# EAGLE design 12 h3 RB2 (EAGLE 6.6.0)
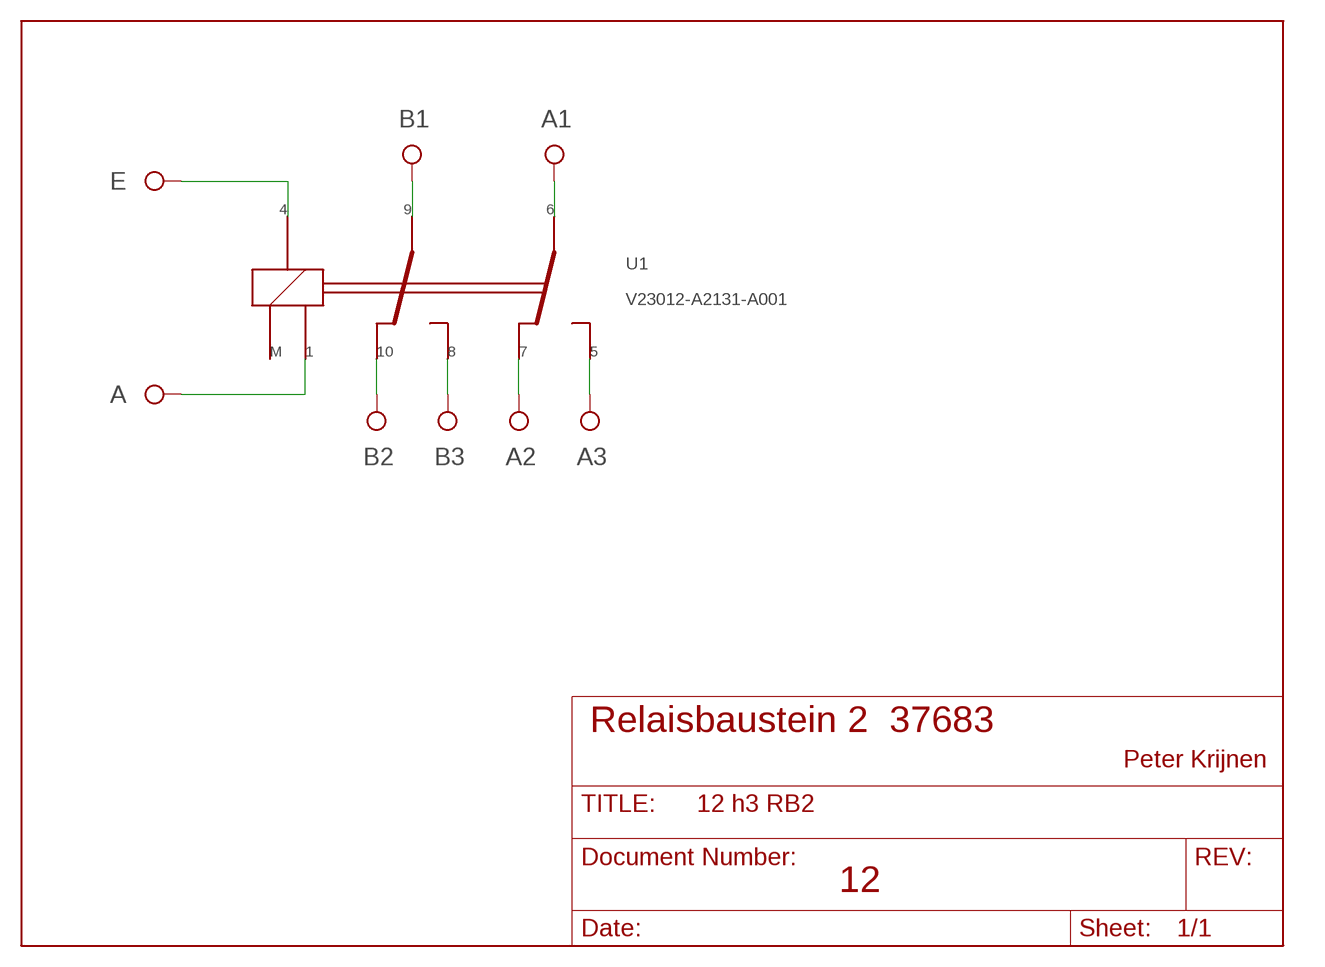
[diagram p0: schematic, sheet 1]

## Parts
A  PIN_2  [PIN_2]
A1  PIN_2  [PIN_2]
A2  PIN_2  [PIN_2]
A3  PIN_2  [PIN_2]
B1  PIN_2  [PIN_2]
B2  PIN_2  [PIN_2]
B3  PIN_2  [PIN_2]
E  PIN_2  [PIN_2]
U1  V23012-A2131-A001  V23012-A2131  [V23012]

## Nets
N$1: B2.P$1 U1.10
N$2: B3.P$1 U1.8
N$3: A2.P$1 U1.7
N$4: A3.P$1 U1.5
N$5: A1.P$1 U1.6
N$6: B1.P$1 U1.9
N$9: A.P$1 U1.1
N$12: E.P$1 U1.4
Unconnected: U1.M

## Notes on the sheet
- Relaisbaustein 2  37683
- Peter Krijnen
- 12

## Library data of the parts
A A1-A3 B1-B3 E = ft_spec:PIN_2
U1 = FT-SPEC:V23012

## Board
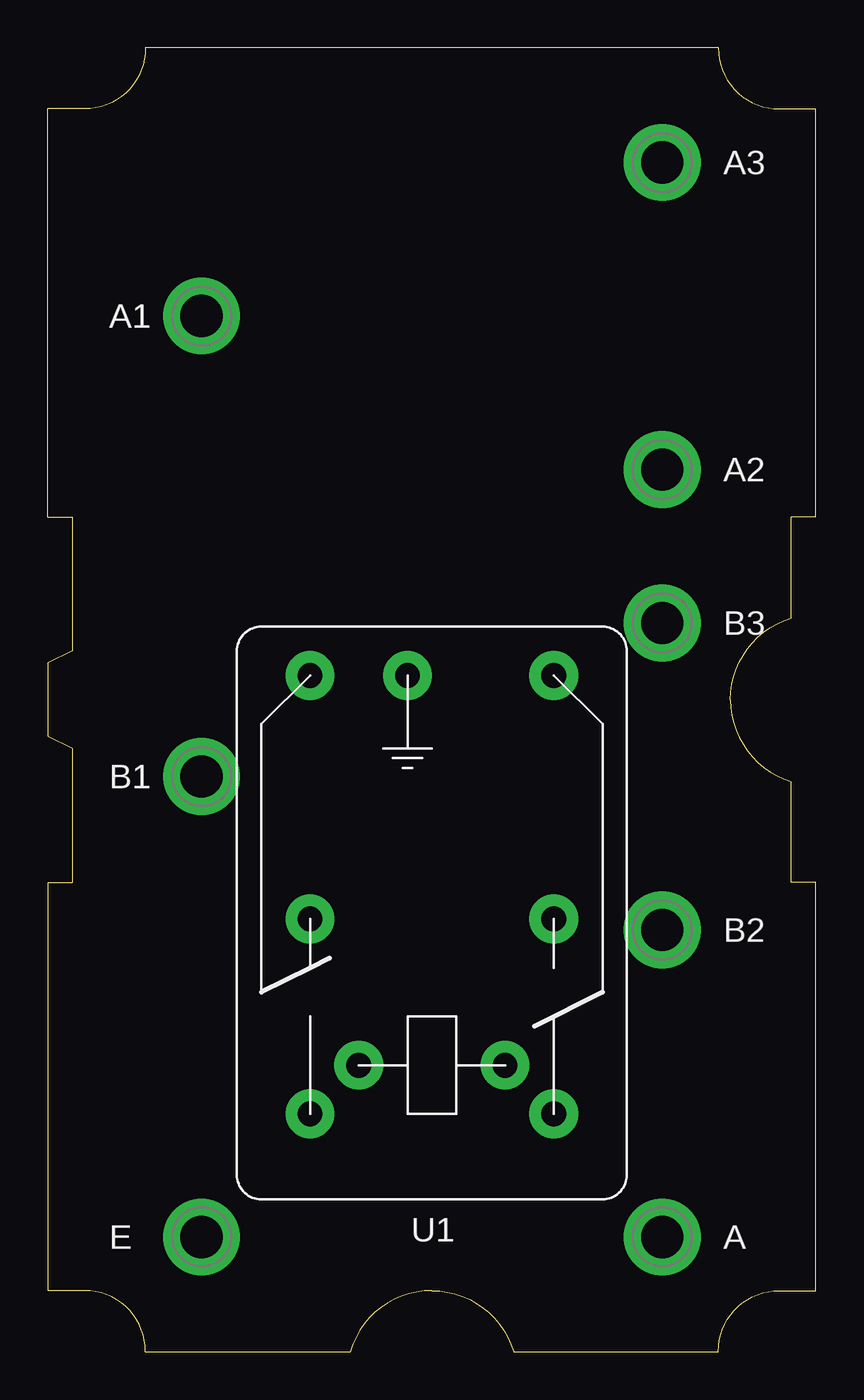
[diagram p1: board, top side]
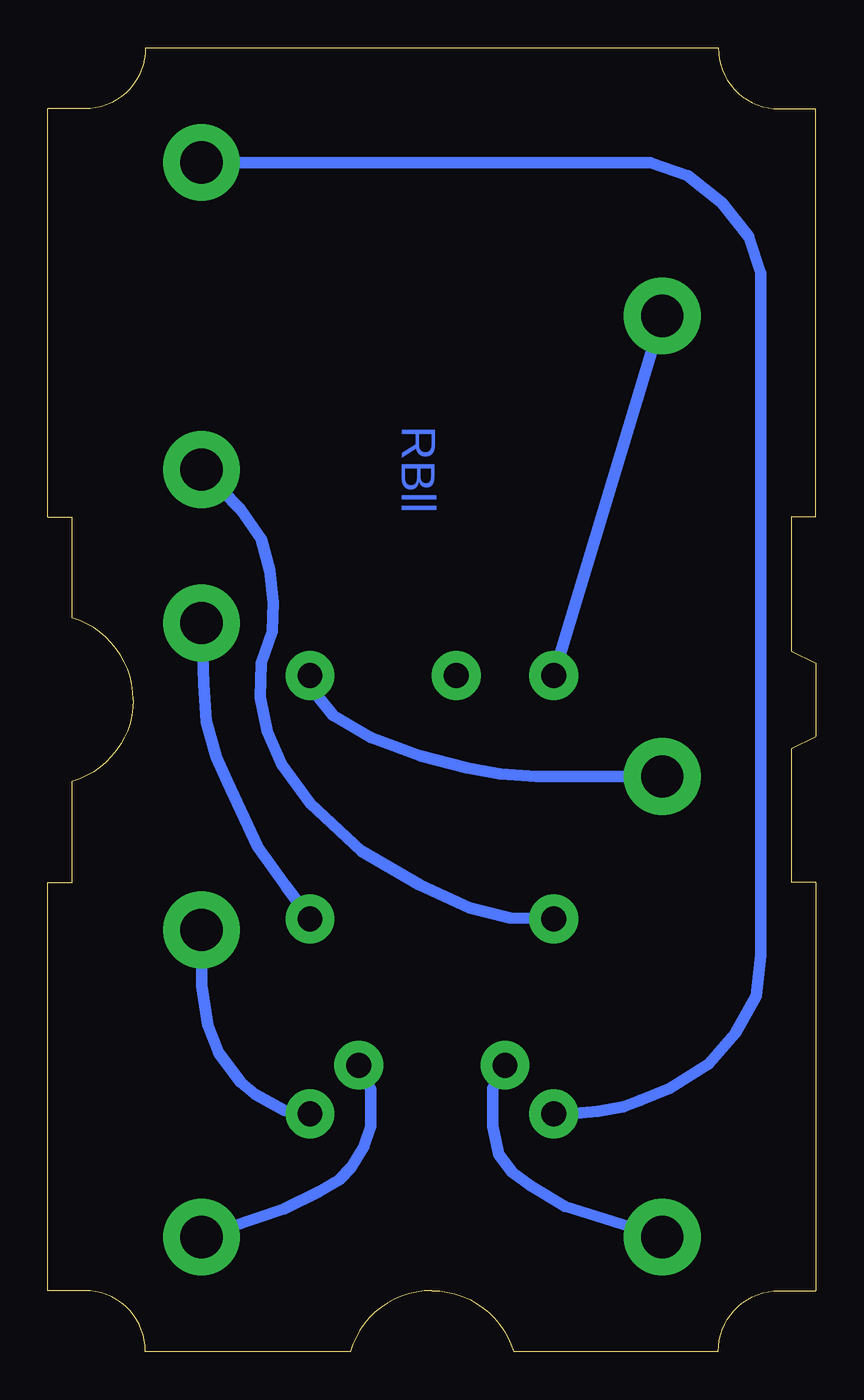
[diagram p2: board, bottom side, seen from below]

Size 40.01 x 67.94 mm. Coordinates in mm from the lower left corner, seen from the top.
Copper layers 16: Bottom 0.035mm
Design rules "default": minimum track width 10mil, minimum drill 24mil, track to track 8mil, track to pad 8mil, pad to pad 8mil, via to via 8mil, smd to smd 8mil, copper to edge 0.25mm, drill to drill 8mil, minimum pad ring 10mil, minimum via ring 8mil, stop-mask expansion 0mil, vias tented up to drill 0mil, thermal gap 10mil

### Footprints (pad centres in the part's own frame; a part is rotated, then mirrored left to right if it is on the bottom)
PIN_2 = drill 2.2 pad 4: P$1 0,0
V23012 = drill 1.3 pad 2.54: 1 -7.62,-3.81; 4 -7.62,3.81; 5 -10.16,6.35; 6 12.7,6.35; 7 0,6.35; 8 0,-6.35; 9 12.7,-6.35; 10 -10.16,-6.35; M 12.7,1.27

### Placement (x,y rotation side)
A  32,5.97 0 top
A1  8,53.98 0 top
A2  32,45.97 0 top
A3  32,61.98 0 top
B1  8,29.97 0 top
B2  32,21.97 0 top
B3  32,37.97 0 top
E  8,5.97 0 top
U1  20,22.54 90 top
U$1  [PRINTFORM_4575]  40.01,0 90 top
U$2  [DIM_4070]  40.01,0 90 top

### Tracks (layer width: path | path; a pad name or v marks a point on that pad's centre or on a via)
N$1
  Bottom 0.61: U1.10 27.69,12.57 29.21,13.4 29.97,14.03 31.11,15.56 31.69,17.02 32,19.05 B2.P$1
N$2
  Bottom 0.61: U1.8 27.62,24.26 29.08,26.29 30.67,29.72 31.24,30.99 31.75,32.83 31.88,34.8 B3.P$1
N$3
  Bottom 0.61: U1.7 15.94,22.61 18.03,23.11 20.64,24.32 23.69,26.1 26.35,28.57 27.81,30.61 28.57,32.32 28.96,34.1 28.89,35.88 28.32,37.53 28.26,39.05 28.45,40.7 28.89,42.35 29.97,43.88 A2.P$1
N$4
  Bottom 0.61: U1.5 12.26,12.45 11.37,12.51 10.03,12.76 9.14,13.08 7.62,13.72 5.59,14.99 4.19,16.57 3.11,18.54 2.86,20.64 2.86,56.2 3.49,58.1 4.89,59.88 6.67,61.28 8.64,61.98 A3.P$1
N$5
  Bottom 0.61: U1.6 A1.P$1
N$6
  Bottom 0.61: U1.9 25.91,34.1 25.15,33.15 23.18,32 20.57,31.05 18.16,30.42 16.45,30.1 14.54,29.97 B1.P$1
N$9
  Bottom 0.61: U1.1 23.18,13.65 23.18,11.75 23.56,10.67 24.19,9.59 24.83,8.95 25.91,8.32 27.69,7.43 A.P$1
N$12
  Bottom 0.61: U1.4 16.83,13.72 16.83,11.75 16.51,10.29 15.81,9.34 14.86,8.64 13.08,7.56 E.P$1

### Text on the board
Bottom: RBll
